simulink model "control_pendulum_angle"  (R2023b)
settings: Solver=FixedStepDiscrete  StartTime=0.0  StopTime=sim_stop_time  FixedStep=FRE_time_step  RelTol=1e-3  EnableMultiTasking=on
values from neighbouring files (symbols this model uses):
  dphi_gain = 0.0    [antisway_with_Quanser.sldd]
  dtheta_gain = 0.0    [antisway_with_Quanser.sldd]
  phi_gain = 0.0    [antisway_with_Quanser.sldd]
  theta_gain = 0.0    [antisway_with_Quanser.sldd]

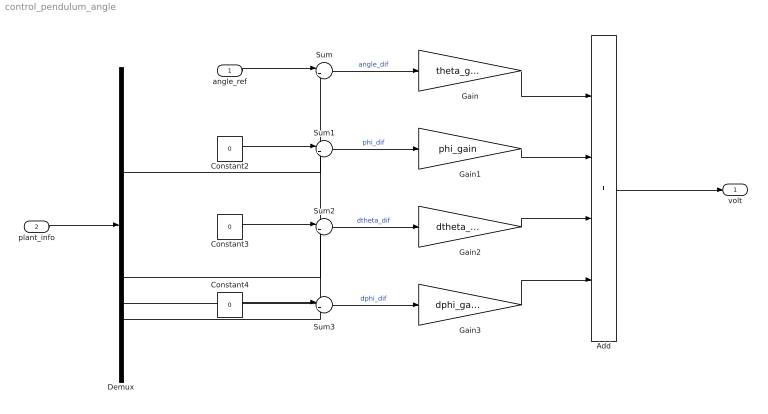
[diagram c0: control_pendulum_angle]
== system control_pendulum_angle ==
  angle_ref : Inport
  plant_info : Inport  Port=2  OutDataTypeStr=single  PortDimensions=4
  Add : Sum  Inputs=++++
  Constant2 : Constant  Value=0  OutDataTypeStr=single
  Constant3 : Constant  Value=0  OutDataTypeStr=single
  Constant4 : Constant  Value=0  OutDataTypeStr=single
  Demux : Demux
  Gain : Gain  Gain=theta_gain
  Gain1 : Gain  Gain=phi_gain
  Gain2 : Gain  Gain=dtheta_gain
  Gain3 : Gain  Gain=dphi_gain
  Sum{,1..3} (4 alike) : Sum  Inputs=|+-
  volt : Outport
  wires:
  plant_info/1 -> Demux/1
  Gain1/1 -> Add/2
  Gain2/1 -> Add/3
  Gain/1 -> Add/1
  Add/1 -> volt/1
  Gain3/1 -> Add/4
  Demux/2 -> Sum1/2
  Sum/1 -> Gain/1  "angle_dif"
  Constant2/1 -> Sum1/1
  Constant3/1 -> Sum2/1
  Demux/3 -> Sum2/2
  angle_ref/1 -> Sum/1
  Demux/4 -> Sum3/2
  Demux/1 -> Sum/2
  Constant4/1 -> Sum3/1
  Sum1/1 -> Gain1/1  "phi_dif"
  Sum2/1 -> Gain2/1  "dtheta_dif"
  Sum3/1 -> Gain3/1  "dphi_dif"
